DATA_BLOCK "RIC_TRANS"
TITLE =
VERSION : 0.1


  STRUCT
   CH1_R1 : REAL ;	//angolo ini start chiusura
   CH1_R2 : REAL ;	//angolo start salita
   CH1_R3 : REAL ;	//angolo start traslazione avanti
   CH1_R4 : REAL ;	//angolo start discesa
   CH1_R5 : REAL ;	//angolo start apertura
   CH1_R6 : REAL ;	//angolo start traslazione indietro
   CH1_R10 : REAL ;	//quota X indietro
   CH1_R11 : REAL ;	//quota X avanti
   CH1_R20 : REAL ;	//quota Y aperto
   CH1_R21 : REAL ;	//quota Y chiuso
   CH1_R23 : REAL ;	//posizione Y in fuoringombro
   CH1_R30 : REAL ;	//quota Z basso
   CH1_R31 : REAL ;	//quota Z alto
   CH1_R33 : REAL ;	//posizione Z in fuoringombro
   CH1_R41 : REAL ;	//anticipo chiusura
   CH1_R42 : REAL ;	//anticipo salita
   CH1_R43 : REAL ;	//anticipo traslaz.av
   CH1_R44 : REAL ;	//anticipo discesa
   CH1_R45 : REAL ;	//anticipo apertura
   CH1_R46 : REAL ;	//anticipo traslaz.ind
   CH1_R47 : REAL ;	//anticipo chiusura manine
   CH1_R48 : REAL ;	//angolo funz_aux fronte on
   CH1_R51 : REAL ;	//angolo funz_aux fronte on
   CH1_R52 : REAL ;	//angolo funz_aux fronte off
   CH1_R53 : REAL ;	//angolo funz_aux retro on
   CH1_R54 : REAL ;	//angolo funz_aux retro off
   CH1_R5D1 : REAL ;
   CH1_R5D2 : REAL ;
   CH1_R5D3 : REAL ;
   CH1_R5D4 : REAL ;
   CH1_R5D5 : REAL ;
   AB_CTR_PR_ANT1 : BOOL ;
   AB_CTR_PR_ANT2 : BOOL ;
   AB_CTR_PR_ANT3 : BOOL ;
   AB_CTR_PR_ANT4 : BOOL ;
   AB_CTR_PR_ANT5 : BOOL ;
   AB_CTR_PR_ANT6 : BOOL ;
   AB_CTR_PR_ANT7 : BOOL ;
   AB_CTR_PR_ANT8 : BOOL ;
   AB_CTR_PR_ANT9 : BOOL ;
   AB_CTR_PR_ANT10 : BOOL ;
   AB_CTR_PR_ANT11 : BOOL ;
   AB_CTR_PR_ANT12 : BOOL ;
   AB_CTR_PR_ANT13 : BOOL ;
   AB_CTR_PR_ANT14 : BOOL ;
   AB_CTR_PR_ANT15 : BOOL ;
   AB_CTR_PR_ANT16 : BOOL ;
   AB_CTR_PR_POST1 : BOOL ;
   AB_CTR_PR_POST2 : BOOL ;
   AB_CTR_PR_POST3 : BOOL ;
   AB_CTR_PR_POST4 : BOOL ;
   AB_CTR_PR_POST5 : BOOL ;
   AB_CTR_PR_POST6 : BOOL ;
   AB_CTR_PR_POST7 : BOOL ;
   AB_CTR_PR_POST8 : BOOL ;
   AB_CTR_PR_POST9 : BOOL ;
   AB_CTR_PR_POST10 : BOOL ;
   AB_CTR_PR_POST11 : BOOL ;
   AB_CTR_PR_POST12 : BOOL ;
   AB_CTR_PR_POST13 : BOOL ;
   AB_CTR_PR_POST14 : BOOL ;
   AB_CTR_PR_POST15 : BOOL ;
   AB_CTR_PR_POST16 : BOOL ;
  END_STRUCT ;
BEGIN
   CH1_R1 := 0.000000e+000;
   CH1_R2 := 0.000000e+000;
   CH1_R3 := 0.000000e+000;
   CH1_R4 := 0.000000e+000;
   CH1_R5 := 0.000000e+000;
   CH1_R6 := 0.000000e+000;
   CH1_R10 := 0.000000e+000;
   CH1_R11 := 0.000000e+000;
   CH1_R20 := 0.000000e+000;
   CH1_R21 := 0.000000e+000;
   CH1_R23 := 0.000000e+000;
   CH1_R30 := 0.000000e+000;
   CH1_R31 := 0.000000e+000;
   CH1_R33 := 0.000000e+000;
   CH1_R41 := 0.000000e+000;
   CH1_R42 := 0.000000e+000;
   CH1_R43 := 0.000000e+000;
   CH1_R44 := 0.000000e+000;
   CH1_R45 := 0.000000e+000;
   CH1_R46 := 0.000000e+000;
   CH1_R47 := 0.000000e+000;
   CH1_R48 := 0.000000e+000;
   CH1_R51 := 0.000000e+000;
   CH1_R52 := 0.000000e+000;
   CH1_R53 := 0.000000e+000;
   CH1_R54 := 0.000000e+000;
   CH1_R5D1 := 0.000000e+000;
   CH1_R5D2 := 0.000000e+000;
   CH1_R5D3 := 0.000000e+000;
   CH1_R5D4 := 0.000000e+000;
   CH1_R5D5 := 0.000000e+000;
   AB_CTR_PR_ANT1 := FALSE;
   AB_CTR_PR_ANT2 := FALSE;
   AB_CTR_PR_ANT3 := FALSE;
   AB_CTR_PR_ANT4 := FALSE;
   AB_CTR_PR_ANT5 := FALSE;
   AB_CTR_PR_ANT6 := FALSE;
   AB_CTR_PR_ANT7 := FALSE;
   AB_CTR_PR_ANT8 := FALSE;
   AB_CTR_PR_ANT9 := FALSE;
   AB_CTR_PR_ANT10 := FALSE;
   AB_CTR_PR_ANT11 := FALSE;
   AB_CTR_PR_ANT12 := FALSE;
   AB_CTR_PR_ANT13 := FALSE;
   AB_CTR_PR_ANT14 := FALSE;
   AB_CTR_PR_ANT15 := FALSE;
   AB_CTR_PR_ANT16 := FALSE;
   AB_CTR_PR_POST1 := FALSE;
   AB_CTR_PR_POST2 := FALSE;
   AB_CTR_PR_POST3 := FALSE;
   AB_CTR_PR_POST4 := FALSE;
   AB_CTR_PR_POST5 := FALSE;
   AB_CTR_PR_POST6 := FALSE;
   AB_CTR_PR_POST7 := FALSE;
   AB_CTR_PR_POST8 := FALSE;
   AB_CTR_PR_POST9 := FALSE;
   AB_CTR_PR_POST10 := FALSE;
   AB_CTR_PR_POST11 := FALSE;
   AB_CTR_PR_POST12 := FALSE;
   AB_CTR_PR_POST13 := FALSE;
   AB_CTR_PR_POST14 := FALSE;
   AB_CTR_PR_POST15 := FALSE;
   AB_CTR_PR_POST16 := FALSE;
END_DATA_BLOCK

